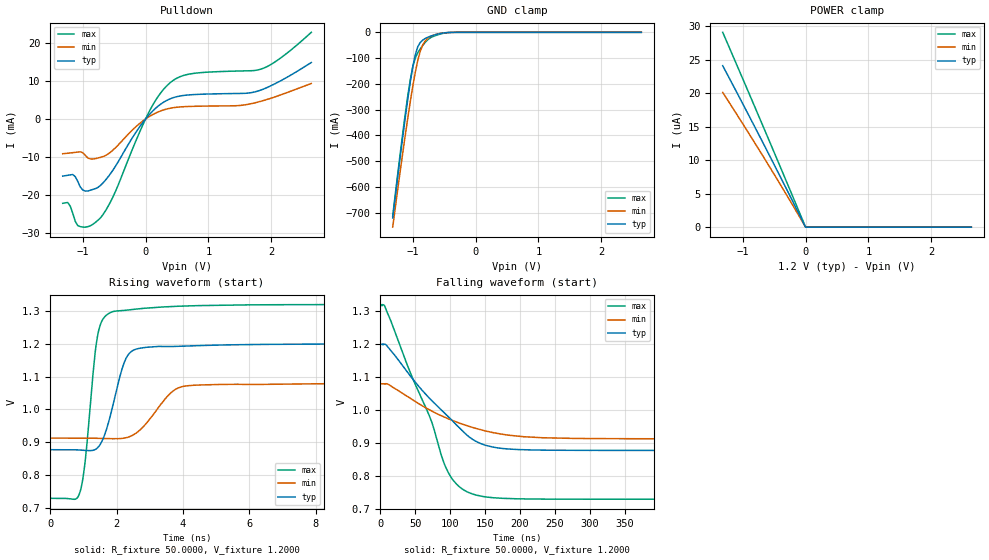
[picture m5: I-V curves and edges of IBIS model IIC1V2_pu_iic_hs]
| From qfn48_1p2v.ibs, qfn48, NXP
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[Model] IIC1V2_pu_iic_hs
|   Model IIC1V2_pu_iic_hs
| This model was characterised for following simulation conditions:
| External (pad) voltage:
|   - Typ: 1.2V,   - Min: 1.08V,   - Max: 1.32V
| Library cells for typ/min/max conditions are connected as defined below:
|  IO - External Pad
|  A - Core Input
|  EN - Output Buffer Enable
|  BOOST - vdde
|  ECS - gnd
|  EGP - gnd
|  ENZI - vdd
|  EPD - gnd
|  EPUN - gnd
|  ZI - NC
|  ZIF - NC
|  gnd - gnd
|  gnde - gnde
|  vdd - vdd
|  vdde - vdde
| All other pins connected to ground
Model_type I/O_open_drain
Polarity   Non-Inverting
Enable   Active-Low
Vinl =   0.5400V
Vinh =   1.2600V
Vmeas =  0.9000V
Cref =   0.0F
Rref =   1.0000k
Vref =   1.2000V
C_comp   3.6136pF   3.4731pF   3.7402pF
|C_comp_pullup   0.9309pF   0.8909pF   0.9450pF
|C_comp_pulldown   2.3305pF   2.4839pF   2.1848pF
[Model Spec]
| variable   typ   min   max
Vinh   0.3600V   0.3240V   0.3960V
Vinl   0.8400V   0.7560V   0.9240V
Vmeas   0.6000V   0.5400V   0.6600V
Vref   1.2000V   1.0800V   1.3200V
Cref   0.0F   0.0F   0.0F
Rref   1.0000k   1.0000k   1.0000k
[Temperature Range]   25.0000   0.1250k   -40.0000
[Voltage Range]   1.2000V   1.0800V   1.3200V
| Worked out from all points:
|   slope of the pulldown table from 0 to 0.18 V, typ, clamps not added: 58.3 ohm
|   GND clamp passes 1 mA (typ) near -0.45 V on its own axis
|   rising waveform, R_fixture 50.0000, V_fixture 1.2000: 20-80 % time 501ps typ, 801ps min, 332ps max; typ from 0.877 V to 1.2 V
|   falling waveform, R_fixture 50.0000, V_fixture 1.2000: 20-80 % time 83.4ns typ, 98.9ns min, 62.7ns max; typ from 1.2 V to 0.877 V
[Pulldown]
|Voltage   I(typ)   I(min)   I(max)
-1.32V    -14.96mA   -9.099mA   -22.09mA
-1.24V    -14.75mA   -8.982mA   -21.89mA
-1.16V    -14.56mA   -8.83mA    -24.7mA
-1.04V    -17.82mA   -8.609mA   -28.21mA
-920mV    -18.88mA   -10.21mA   -28.21mA
-720mV    -17.44mA   -10.07mA   -25.94mA
-520mV    -13.41mA   -8.157mA   -20.44mA
80mV      1.521mA    840uA      2.628mA
440mV     5.569mA    2.951mA    10.1mA
760mV     6.377mA    3.307mA    11.92mA
1.84V     7.592mA    4.649mA    13.07mA
2.64V     14.79mA    9.288mA    22.7mA
[GND_clamp]
|Voltage   I(typ)   I(min)   I(max)
-1.32V    -720.7mA   -756.5mA   -713.8mA
-1.12V    -330.9mA   -399.5mA   -316.8mA
-1.04V    -192.5mA   -269.2mA   -184.5mA
-1V       -133.6mA   -209.3mA   -133.5mA
-960mV    -86.76mA   -154.8mA   -99.49mA
-920mV    -55.71mA   -108.2mA   -79.05mA
-880mV    -39.04mA   -72.36mA   -63.74mA
-840mV    -29.93mA   -48.01mA   -50.29mA
-760mV    -18.95mA   -23.41mA   -28.35mA
-640mV    -9.243mA   -8.645mA   -12.76mA
-400mV    -357.8uA   -419.3uA   -472.1uA
2.64V     0A         0A         0A
[POWER_clamp]
|Voltage   I(typ)   I(min)   I(max)
-1.32V    24.09uA    20.1uA     29.06uA
-640mV    11.88uA    10.01uA    14.23uA
0V        86.89pA    4.342nA    7.851pA
2.64V     0A         0A         0A
[Ramp]
| variable   typ   min   max
dV/dt_r  0.1939/0.5012n   0.1006/0.8013n   0.3549/0.3321n
dV/dt_f  0.1938/83.3790n   0.1006/98.8796n   0.3549/62.6680n
R_load = 50.0000
[Rising Waveform]
R_fixture= 50.0000
V_fixture= 1.2000
V_fixture_min= 1.0800
V_fixture_max= 1.3200
|time   V(typ)   V(min)   V(max)
0s        876.9mV    912.3mV    728.5mV
906.6ps   875.9mV    912.4mV    751.2mV
1.061ns   874.8mV    912.4mV    850.1mV
1.38ns    879mV      911.8mV    1.195V
1.66ns    928.6mV    911.1mV    1.285V
2.167ns   1.125V     911.4mV    1.301V
2.48ns    1.179V     920.9mV    1.305V
3.848ns   1.192V     1.065V     1.315V
6.133ns   1.198V     1.076V     1.319V
1us       1.2V       1.08V      1.32V
[Falling Waveform]
R_fixture= 50.0000
V_fixture= 1.2000
V_fixture_min= 1.0800
V_fixture_max= 1.3200
|time   V(typ)   V(min)   V(max)
0s        1.2V       1.08V      1.32V
6.276ns   1.2V       1.08V      1.317V
41.07ns   1.109V     1.038V     1.124V
69.4ns    1.038V     1.002V     987.2mV
95.68ns   983.4mV    975mV      817.1mV
113.7ns   945mV      960.1mV    765.8mV
137ns     904.9mV    944.2mV    741.6mV
174.7ns   883.3mV    926.5mV    731.7mV
267.1ns   877.7mV    914.1mV    729.1mV
1us       877mV      912.4mV    728.6mV
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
